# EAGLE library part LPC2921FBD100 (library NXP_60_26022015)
ARM9 microcontroller with CAN, LIN, and USB The LPC2921/2923/2925 combine an ARM968E-S CPU core with two integrated TCM blocks operating at frequencies of up to 125 MHz, Full-speed USB 2.0 device controller, CAN and LIN, up to 40 kB SRAM, up to 512 kB flash memory, two 10-bit ADCs, and multiple serial and parallel interfaces in a single chip targeted at consumer, industrial, and communication markets. To optimize system power consumption, the LPC2921/2923/2925 has a very flexible Clock Generation Unit (CGU) that provides dynamic clock gating and scaling. AAL Eindhoven MK
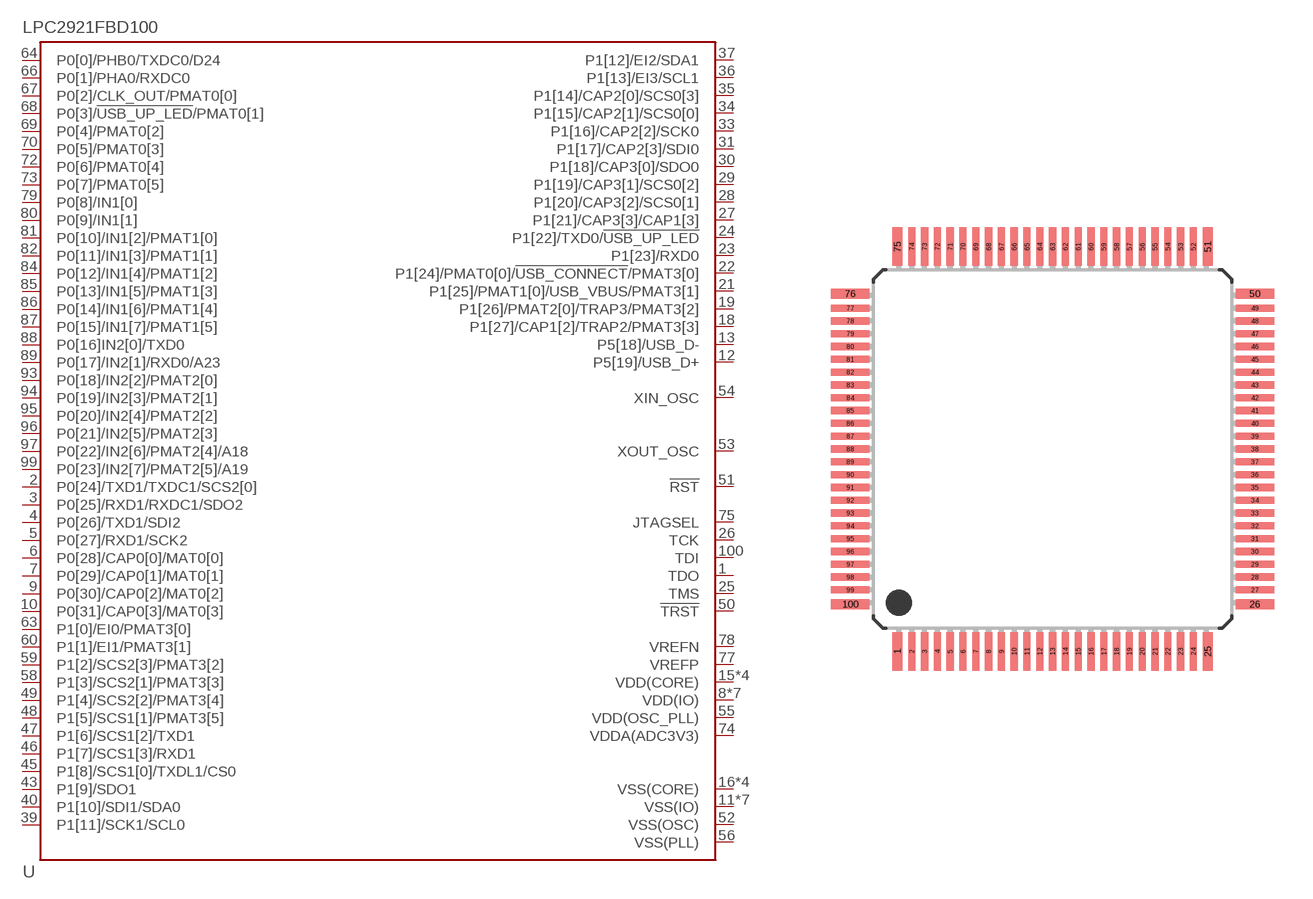
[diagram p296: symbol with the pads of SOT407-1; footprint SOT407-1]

Designator prefix U

## LPC2921FBD100 (FLASH: 128kB; SRAM: 24kB)  [SOT407-1]
1  TDO
2  P0[24]/TXD1/TXDC1/SCS2[0]
3  P0[25]/RXD1/RXDC1/SDO2
4  P0[26]/TXD1/SDI2
5  P0[27]/RXD1/SCK2
6  P0[28]/CAP0[0]/MAT0[0]
7  P0[29]/CAP0[1]/MAT0[1]
8  VDD(IO)
9  P0[30]/CAP0[2]/MAT0[2]
10  P0[31]/CAP0[3]/MAT0[3]
11  VSS(IO)
12  P5[19]/USB_D+
13  P5[18]/USB_D-
14  VDD(IO)
15  VDD(CORE)
16  VSS(CORE)
17  VSS(IO)
18  P1[27]/CAP1[2]/TRAP2/PMAT3[3]
19  P1[26]/PMAT2[0]/TRAP3/PMAT3[2]
20  VDD(IO)
21  P1[25]/PMAT1[0]/USB_VBUS/PMAT3[1]
22  P1[24]/PMAT0[0]/!USB_CONNECT!/PMAT3[0]
23  P1[23]/RXD0
24  P1[22]/TXD0/!USB_UP_LED!
25  TMS
26  TCK
27  P1[21]/CAP3[3]/CAP1[3]
28  P1[20]/CAP3[2]/SCS0[1]
29  P1[19]/CAP3[1]/SCS0[2]
30  P1[18]/CAP3[0]/SDO0
31  P1[17]/CAP2[3]/SDI0
32  VSS(IO)
33  P1[16]/CAP2[2]/SCK0
34  P1[15]/CAP2[1]/SCS0[0]
35  P1[14]/CAP2[0]/SCS0[3]
36  P1[13]/EI3/SCL1
37  P1[12]/EI2/SDA1
38  VDD(IO)
39  P1[11]/SCK1/SCL0
40  P1[10]/SDI1/SDA0
41  VSS(CORE)
42  VDD(CORE)
43  P1[9]/SDO1
44  VSS(IO)
45  P1[8]/SCS1[0]/TXDL1/CS0
46  P1[7]/SCS1[3]/RXD1
47  P1[6]/SCS1[2]/TXD1
48  P1[5]/SCS1[1]/PMAT3[5]
49  P1[4]/SCS2[2]/PMAT3[4]
50  !TRST!
51  !RST!
52  VSS(OSC)
53  XOUT_OSC
54  XIN_OSC
55  VDD(OSC_PLL)
56  VSS(PLL)
57  VDD(IO)
58  P1[3]/SCS2[1]/PMAT3[3]
59  P1[2]/SCS2[3]/PMAT3[2]
60  P1[1]/EI1/PMAT3[1]
61  VSS(CORE)
62  VDD(CORE)
63  P1[0]/EI0/PMAT3[0]
64  P0[0]/PHB0/TXDC0/D24
65  VSS(IO)
66  P0[1]/PHA0/RXDC0
67  P0[2]/CLK_OUT/PMAT0[0]
68  P0[3]/!USB_UP_LED!/PMAT0[1]
69  P0[4]/PMAT0[2]
70  P0[5]/PMAT0[3]
71  VDD(IO)
72  P0[6]/PMAT0[4]
73  P0[7]/PMAT0[5]
74  VDDA(ADC3V3)
75  JTAGSEL
77  VREFP
78  VREFN
79  P0[8]/IN1[0]
80  P0[9]/IN1[1]
81  P0[10]/IN1[2]/PMAT1[0]
82  P0[11]/IN1[3]/PMAT1[1]
83  VSS(IO)
84  P0[12]/IN1[4]/PMAT1[2]
85  P0[13]/IN1[5]/PMAT1[3]
86  P0[14]/IN1[6]/PMAT1[4]
87  P0[15]/IN1[7]/PMAT1[5]
88  P0[16]IN2[0]/TXD0
89  P0[17]/IN2[1]/RXD0/A23
90  VDD(CORE)
91  VSS(CORE)
92  VDD(IO)
93  P0[18]/IN2[2]/PMAT2[0]
94  P0[19]/IN2[3]/PMAT2[1]
95  P0[20]/IN2[4]/PMAT2[2]
96  P0[21]/IN2[5]/PMAT2[3]
97  P0[22]/IN2[6]/PMAT2[4]/A18
98  VSS(IO)
99  P0[23]/IN2[7]/PMAT2[5]/A19
100  TDI

## Footprint SOT407-1 (pad centres in mm)
SOT407-1 LQFP100: plastic low profile quad flat package; 100 leads; body 14 x 14 x 1.4 mm JEDEC: MS-026 IEC: 136E20
smd 0.4 x 1.5: 1 -6.06,-7.9; 25 6.06,-7.9; 51 6.06,7.9; 75 -6.06,7.9
smd 0.28 x 1.5: 2 -5.5,-7.9; 3 -5,-7.9; 4 -4.5,-7.9; 5 -4,-7.9; 6 -3.5,-7.9; 7 -3,-7.9; 8 -2.5,-7.9; 9 -2,-7.9; 10 -1.5,-7.9; 11 -1,-7.9; 12 -0.5,-7.9; 13 0,-7.9; 14 0.5,-7.9; 15 1,-7.9; 16 1.5,-7.9; 17 2,-7.9; 18 2.5,-7.9; 19 3,-7.9; 20 3.5,-7.9; 21 4,-7.9; 22 4.5,-7.9; 23 5,-7.9; 24 5.5,-7.9; 52 5.5,7.9; 53 5,7.9; 54 4.5,7.9; 55 4,7.9; 56 3.5,7.9; 57 3,7.9; 58 2.5,7.9; 59 2,7.9; 60 1.5,7.9; 61 1,7.9; 62 0.5,7.9; 63 0,7.9; 64 -0.5,7.9; 65 -1,7.9; 66 -1.5,7.9; 67 -2,7.9; 68 -2.5,7.9; 69 -3,7.9; 70 -3.5,7.9; 71 -4,7.9; 72 -4.5,7.9; 73 -5,7.9; 74 -5.5,7.9
smd 1.5 x 0.4: 26 7.9,-6.06; 50 7.9,6.06; 76 -7.9,6.06; 100 -7.9,-6.06
smd 1.5 x 0.28: 27 7.9,-5.5; 28 7.9,-5; 29 7.9,-4.5; 30 7.9,-4; 31 7.9,-3.5; 32 7.9,-3; 33 7.9,-2.5; 34 7.9,-2; 35 7.9,-1.5; 36 7.9,-1; 37 7.9,-0.5; 38 7.9,0; 39 7.9,0.5; 40 7.9,1; 41 7.9,1.5; 42 7.9,2; 43 7.9,2.5; 44 7.9,3; 45 7.9,3.5; 46 7.9,4; 47 7.9,4.5; 48 7.9,5; 49 7.9,5.5; 77 -7.9,5.5; 78 -7.9,5; 79 -7.9,4.5; 80 -7.9,4; 81 -7.9,3.5; 82 -7.9,3; 83 -7.9,2.5; 84 -7.9,2; 85 -7.9,1.5; 86 -7.9,1; 87 -7.9,0.5; 88 -7.9,0; 89 -7.9,-0.5; 90 -7.9,-1; 91 -7.9,-1.5; 92 -7.9,-2; 93 -7.9,-2.5; 94 -7.9,-3; 95 -7.9,-3.5; 96 -7.9,-4; 97 -7.9,-4.5; 98 -7.9,-5; 99 -7.9,-5.5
